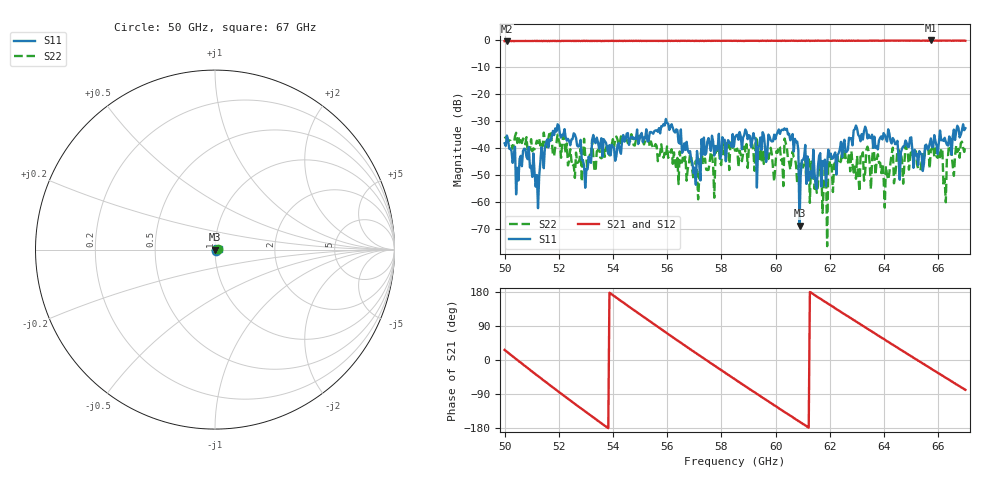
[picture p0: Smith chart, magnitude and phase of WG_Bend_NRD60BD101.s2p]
!Agilent Technologies,E8361A,US42410132,A.06.03.05
!Agilent E8361A: A.06.03.05
!Date: Friday, July 11, 2008 17:09:08
!Correction: S11(Full 2 Port(1,2)) S21(Full 2 Port(1,2)) S12(Full 2 Port(1,2)) S22(Full 2 Port(1,2))
!S2P File: Measurements: S11, S21, S12, S22:
# Hz S  MA  R 50
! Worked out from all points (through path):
!   401 points, 50 GHz to 67 GHz, reference 50 ohm
!   highest |S21| = -0.35 dB at 65.72 GHz (marker M1); lowest = -0.7 dB at 50.09 GHz (marker M2)
!   lowest |S11| = -68.7 dB at 60.88 GHz (marker M3), VSWR 1.00, Z = 50 - j0.0214 ohm
!   |S11| at or under -10 dB: start of sweep to end of sweep
!   |S22| runs from -76.2 to -33.8 dB; largest |S21 - S12| = 0.019
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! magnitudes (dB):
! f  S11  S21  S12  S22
! 50 GHz  -38.3  -0.6  -0.5  -36.5
! 50.09 GHz  -35.4  -0.7  -0.5  -36.5
! 50.81 GHz  -43.3  -0.6  -0.6  -36.0
! 51.19 GHz  -50.0  -0.5  -0.5  -37.3
! 51.91 GHz  -33.9  -0.6  -0.5  -38.1
! 52.85 GHz  -44.4  -0.5  -0.5  -52.3
! 55.7 GHz  -32.7  -0.5  -0.5  -43.4
! 56.29 GHz  -34.3  -0.5  -0.4  -45.3
! 56.97 GHz  -49.3  -0.5  -0.5  -51.6
! 58.5 GHz  -36.1  -0.5  -0.4  -41.0
! 59.39 GHz  -39.4  -0.6  -0.4  -44.8
! 60.33 GHz  -32.8  -0.4  -0.4  -36.5
! 60.88 GHz  -68.7  -0.5  -0.4  -46.8
! 61.35 GHz  -51.2  -0.5  -0.4  -46.8
! 61.81 GHz  -44.3  -0.4  -0.4  -46.4
! 62.24 GHz  -49.8  -0.5  -0.4  -43.4
! 62.96 GHz  -31.7  -0.4  -0.4  -51.3
! 64.19 GHz  -34.6  -0.4  -0.4  -49.1
! 65.72 GHz  -36.5  -0.4  -0.3  -40.6
! 66.28 GHz  -37.7  -0.4  -0.4  -60.0
! 66.41 GHz  -35.7  -0.4  -0.4  -36.8
! 67 GHz  -32.7  -0.5  -0.5  -39.1
